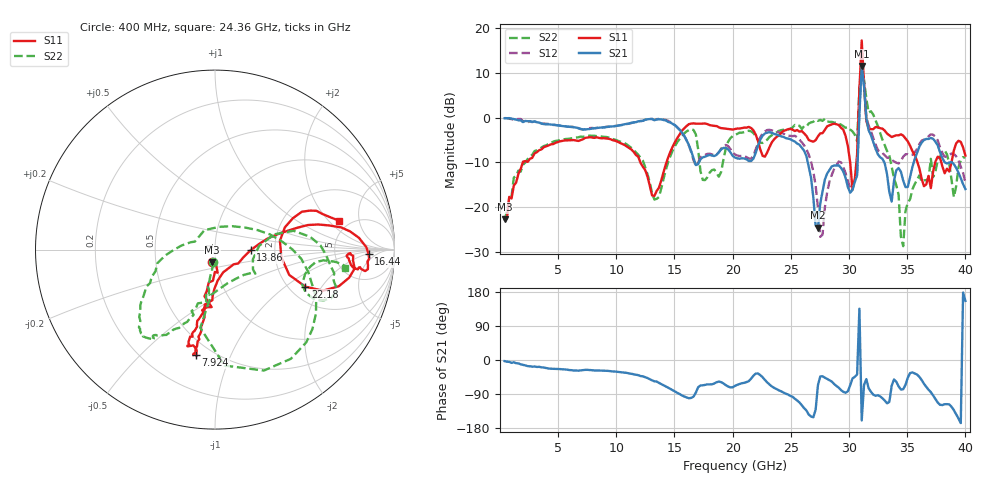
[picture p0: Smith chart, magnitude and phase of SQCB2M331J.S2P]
! Network Analyzer HP8722ES.07.66: Jul 25, 2000 Serial No. US39175408
! 27 Oct 2004  14:19:00
! Frequency  S11  S21  S12  S22
# HZ  S  DB R  50
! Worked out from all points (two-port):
!   201 points, 400 MHz to 40 GHz, reference 50 ohm
!   highest |S21| = 11.56 dB at 31.09 GHz (marker M1); lowest = -24.7 dB at 27.33 GHz (marker M2)
!   |S21| within 3 dB of the highest: 31.03 GHz to 31.22 GHz (188.2 MHz wide, 0.605 % of centre)
!   lowest |S11| = -22.8 dB at 400 MHz (marker M3), VSWR 1.16, Z = 48 - j6.85 ohm
!   |S11| at or under -10 dB: start of sweep to 1.968 GHz; 12.06 GHz to 14.32 GHz (2.253 GHz wide, 17.1 % of centre); 35.88 GHz to 37.41 GHz (1.533 GHz wide, 4.18 % of centre)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
!   |S22| runs from -28.8 to 10.1 dB; largest |S21 - S12| = 0.93
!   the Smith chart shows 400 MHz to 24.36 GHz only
!   S11 on the Smith chart (normalised r, x): 400 MHz: 0.96, -0.14; 7.924 GHz: 0.41, -0.75; 13.86 GHz: 1.49, -0.01; 16.44 GHz: 12, -2; 22.18 GHz: 2.43, -1.43; 24.36 GHz: 4.07, +2.65
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4e8  -22.77 -102.3  -0.15 -2.9  -0.11 -2.5  -23.04 -100.8
7.132e9  -4.85 -100.3  -2.66 -26.7  -2.70 -26.6  -4.32 -125.0
7.924e9  -4.48 -100.2  -2.48 -26.8  -2.33 -25.6  -4.09 -129.7
1.3666e10  -15.70 -15.1  -0.38 -60.4  -0.29 -57.9  -17.79 79.5
1.3864e10  -14.06 -1.1  -0.42 -63.5  -0.33 -61.0  -15.86 54.0
1.6438e10  -1.35 -1.7  -7.55 -100.0  -7.76 -97.0  -2.60 -55.2
1.7428e10  -1.34 -5.7  -8.91 -66.9  -8.51 -62.4  -13.96 -70.1
2.02e10  -2.57 -1.8  -8.96 -68.4  -8.27 -64.2  -3.93 -5.8
2.218e10  -5.28 -22.3  -6.28 -35.6  -5.66 -32.1  -5.04 -25.5
2.4358e10  -2.98 13.2  -4.32 -85.5  -3.57 -80.9  -2.71 -8.2
2.6932e10  -5.40 -156.9  -17.87 -151.1  -12.12 -146.8  -0.94 -16.7
2.7328e10  -4.21 161.5  -24.67 -66.1  -20.20 -147.1  -0.75 -22.6
2.8516e10  -1.53 85.0  -10.94 -56.9  -12.85 -33.7  -0.96 -35.1
2.9506e10  -2.72 28.1  -12.09 -83.8  -11.04 -68.1  -1.92 -41.9
3.0694e10  -8.25 73.6  -12.96 -38.2  -12.64 -27.3  -5.30 -60.6
3.0892e10  6.28 17.4  0.82 135.3  1.93 150.8  6.79 -29.3
3.109e10  17.26 -77.0  11.56 -159.3  11.65 -145.3  10.15 131.2
3.1288e10  7.68 -47.4  7.10 -66.0  7.32 -51.3  8.47 -100.3
3.1486e10  -0.71 -42.4  -0.13 -50.3  0.16 -36.1  4.26 -68.2
3.3466e10  -3.98 -124.4  -16.71 -110.5  -9.04 -71.7  -8.46 -134.1
3.4654e10  -4.04 -147.8  -14.09 -77.1  -8.77 -55.5  -28.79 -44.9
4e10  -8.51 -124.8  -15.99 156.1  -14.57 -141.1  -9.02 -90.1
